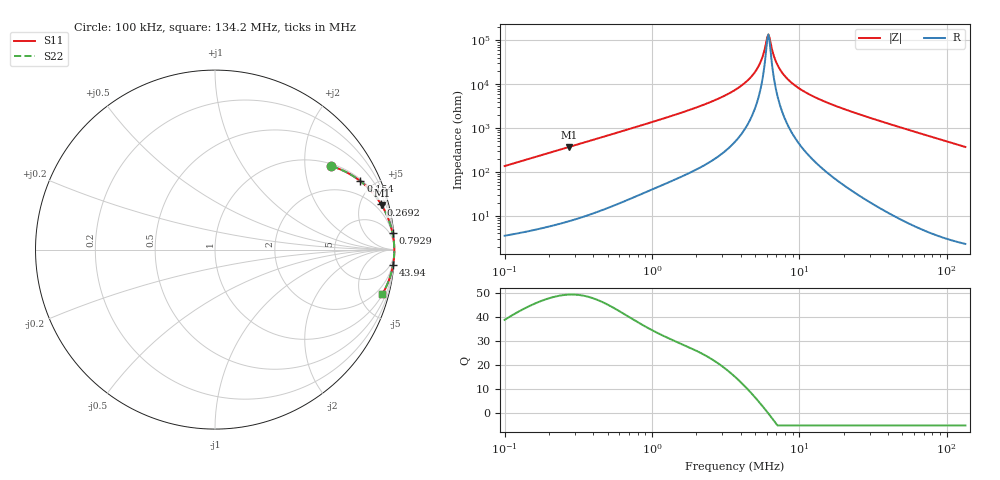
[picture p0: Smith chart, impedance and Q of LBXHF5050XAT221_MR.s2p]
! LBXHF5050XAT221_MR  S-PARAMETER MODEL  ( General Type )
! Model Generated by TAIYO YUDEN Corporation (http://www.ty-top.com)
! Version 1.0
! TAIYO YUDEN Control No. 201105NI43SB-FBB
! Copyright(c) 2020 TAIYO YUDEN CO.,LTD. All Rights Reserved.
! Product Description (link to TY-COMPAS)
! https://ds.yuden.co.jp/TYCOMPAS/or/detail?pn=LBXHF5050XAT221MMR&u=M
! Products Name : Inductors
! Characteristics :
!  Inductance : 220 uH , SRF(min) : 4.0 MHz , DC Resistance(max) : 1.692 Ohm
!  Rated Current : Saturation :380 mA , Temp Rise : 280 mA
!  Case Size : 5.0 x 5.0 / 0.197 x 0.197 [mm/inch] , Thickness : 3.1 / 0.122 [mm/inch]
!  (Conditions: Temperature = 25 degC , DC Bias Current/Voltage = 0A / 0V)
! External Node Assignments :
!  1  o---GGG---o  2
! GND o---------o GND
! Frequency Range : 0.1MHz  -  134.160692MHz  [ 402 STEP ]
# MHz S RI R 50
! Freq[MHz].  S11 Real  S11 Imag  S21 Real  S21 Imag  S12 Real  S12 Imag  S22 Real  S22 Imag
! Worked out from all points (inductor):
!   401 points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, 100 kHz to 134.2 MHz, reference 50 ohm
!   read as one part in series: L = 217 uH near 103.7 kHz
!   highest Q = 49.3 at 274.1 kHz (marker M1), where L = 216 uH
!   self-resonance near 6.064 MHz
!   S11 on the Smith chart (normalised r, x): 100 kHz: 1.07, +2.73; 154 kHz: 1.09, +4.20; 269.2 kHz: 1.15, +7.32; 792.9 kHz: 2, +22; 43.94 MHz: 1, -23; 134.2 MHz: 1.05, -7.45
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0.1  0.6479 0.4649  0.3521 -0.4649  0.3521 -0.4649  0.6479 0.4649
0.154049  0.8098 0.3815  0.1902 -0.3815  0.1902 -0.3815  0.8098 0.3815
0.269184  0.9261 0.2517  0.0739 -0.2517  0.0739 -0.2517  0.9261 0.2517
0.274074  0.9284 0.2478  0.0716 -0.2478  0.0716 -0.2478  0.9284 0.2478
0.334101  0.9499 0.2083  0.0501 -0.2083  0.0501 -0.2083  0.9499 0.2083
0.792852  0.9892 0.0911  0.0108 -0.0911  0.0108 -0.0911  0.9892 0.0911
1.116232  0.9939 0.0643  0.00611 -0.0643  0.00611 -0.0643  0.9939 0.0643
2.377689  0.9981 0.027  0.00188 -0.027  0.00188 -0.027  0.9981 0.027
3.729338  0.999 0.0129  0.00104 -0.0129  0.00104 -0.0129  0.999 0.0129
4.465009  0.9991 0.00809  0.000873 -0.00809  0.000873 -0.00809  0.9991 0.00809
5.064724  0.9992 0.00488  0.000795 -0.00488  0.000795 -0.00488  0.9992 0.00488
5.442921  0.9992 0.00308  0.000763 -0.00308  0.000763 -0.00308  0.9992 0.00308
5.955625  0.9993 0.000858  0.000736 -0.000858  0.000736 -0.000858  0.9993 0.000858
6.173984  0.9993 -3.02e-05  0.000728 3.02e-05  0.000728 3.02e-05  0.9993 -3.02e-05
6.400348  0.9993 -0.000919  0.000723 0.000919  0.000723 0.000919  0.9993 -0.000919
7.003239  0.9993 -0.00315  0.000718 0.00315  0.000718 0.00315  0.9993 -0.00315
7.802132  0.9993 -0.00586  0.000729 0.00586  0.000729 0.00586  0.9993 -0.00586
9.341227  0.9992 -0.0106  0.000789 0.0106  0.000789 0.0106  0.9992 -0.0106
12.23742  0.999 -0.0183  0.000998 0.0183  0.000998 0.0183  0.999 -0.0183
40.88529  0.9929 -0.0795  0.0071 0.0795  0.0071 0.0795  0.9929 -0.0795
43.93831  0.9919 -0.0856  0.00814 0.0856  0.00814 0.0856  0.9919 -0.0856
134.1607  0.9314 -0.2497  0.0686 0.2497  0.0686 0.2497  0.9314 -0.2497
